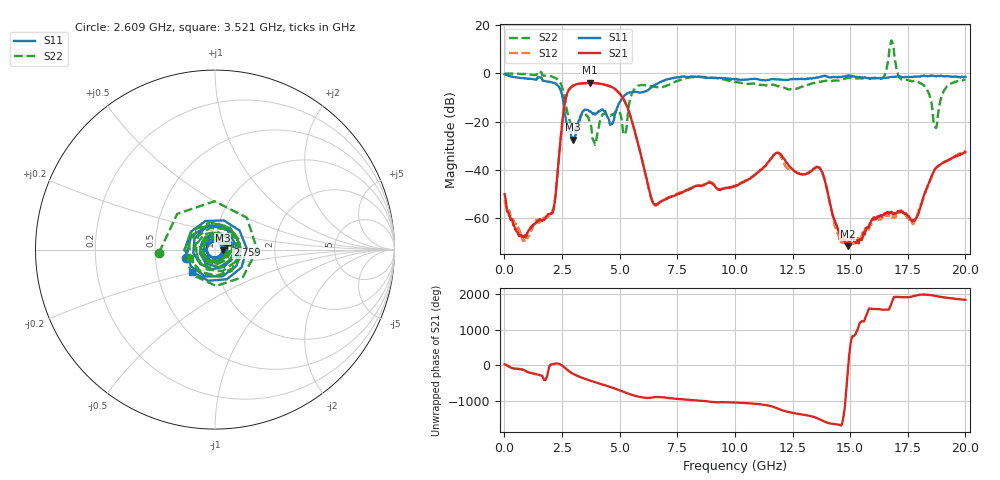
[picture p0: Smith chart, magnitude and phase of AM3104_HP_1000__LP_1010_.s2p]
!Created with skrf (http://scikit-rf.org).
# Hz S RI R 50.0
!freq ReS11 ImS11 ReS21 ImS21 ReS12 ImS12 ReS22 ImS22
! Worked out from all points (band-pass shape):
!   1601 points, 10 MHz to 20 GHz, reference 50 ohm
!   highest |S21| = -3.88 dB at 3.708 GHz (marker M1); lowest = -71.5 dB at 14.9 GHz (marker M2)
!   |S21| within 3 dB of the highest: 2.79 GHz to 4.855 GHz (2.065 GHz wide, 54 % of centre)
!   lowest |S11| = -27.5 dB at 2.984 GHz (marker M3), VSWR 1.09, Z = 54.4 - j0.447 ohm
!   |S11| at or under -10 dB: 2.526 GHz to 5.131 GHz (2.606 GHz wide, 68.1 % of centre)
!   |S22| runs from -29.5 to 13.6 dB; largest |S21 - S12| = 0.051
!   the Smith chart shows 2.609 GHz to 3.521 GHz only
!   S11 on the Smith chart (normalised r, x): 2.609 GHz: 0.72, -0.07; 2.759 GHz: 1.15, +0.06; 3.521 GHz: 0.75, -0.19
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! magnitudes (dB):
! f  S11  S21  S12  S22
! 10 MHz  -0.4  -50.0  -52.5  0.0
! 859.6 MHz  -2.0  -67.5  -68.9  -0.2
! 2.046 GHz  -3.6  -58.0  -57.8  -1.2
! 2.609 GHz  -15.4  -13.1  -13.1  -10.1
! 2.759 GHz  -22.6  -7.5  -7.5  -16.9
! 2.984 GHz  -27.5  -5.0  -5.1  -23.5
! 3.346 GHz  -16.8  -4.1  -4.2  -17.3
! 3.521 GHz  -15.0  -4.0  -4.1  -16.6
! 3.708 GHz  -15.7  -3.9  -3.9  -20.3
! 4.658 GHz  -20.9  -5.6  -5.8  -17.1
! 5.17 GHz  -9.5  -10.6  -10.6  -24.8
! 5.67 GHz  -7.7  -24.4  -24.4  -6.1
! 6.682 GHz  -4.0  -53.8  -54.0  -5.7
! 10.01 GHz  -2.5  -46.7  -46.8  -3.6
! 11.83 GHz  -2.5  -32.9  -32.9  -5.2
! 13.34 GHz  -2.1  -40.3  -40.2  -4.2
! 14.9 GHz  -0.9  -71.5  -70.3  -1.8
! 16.68 GHz  -1.6  -57.8  -59.0  7.2
! 17.78 GHz  -1.3  -60.9  -61.6  -3.1
! 18.69 GHz  -1.1  -39.5  -39.5  -22.1
! 19.14 GHz  -1.2  -36.5  -36.4  -6.2
! 20 GHz  -1.4  -32.6  -32.0  -2.6
